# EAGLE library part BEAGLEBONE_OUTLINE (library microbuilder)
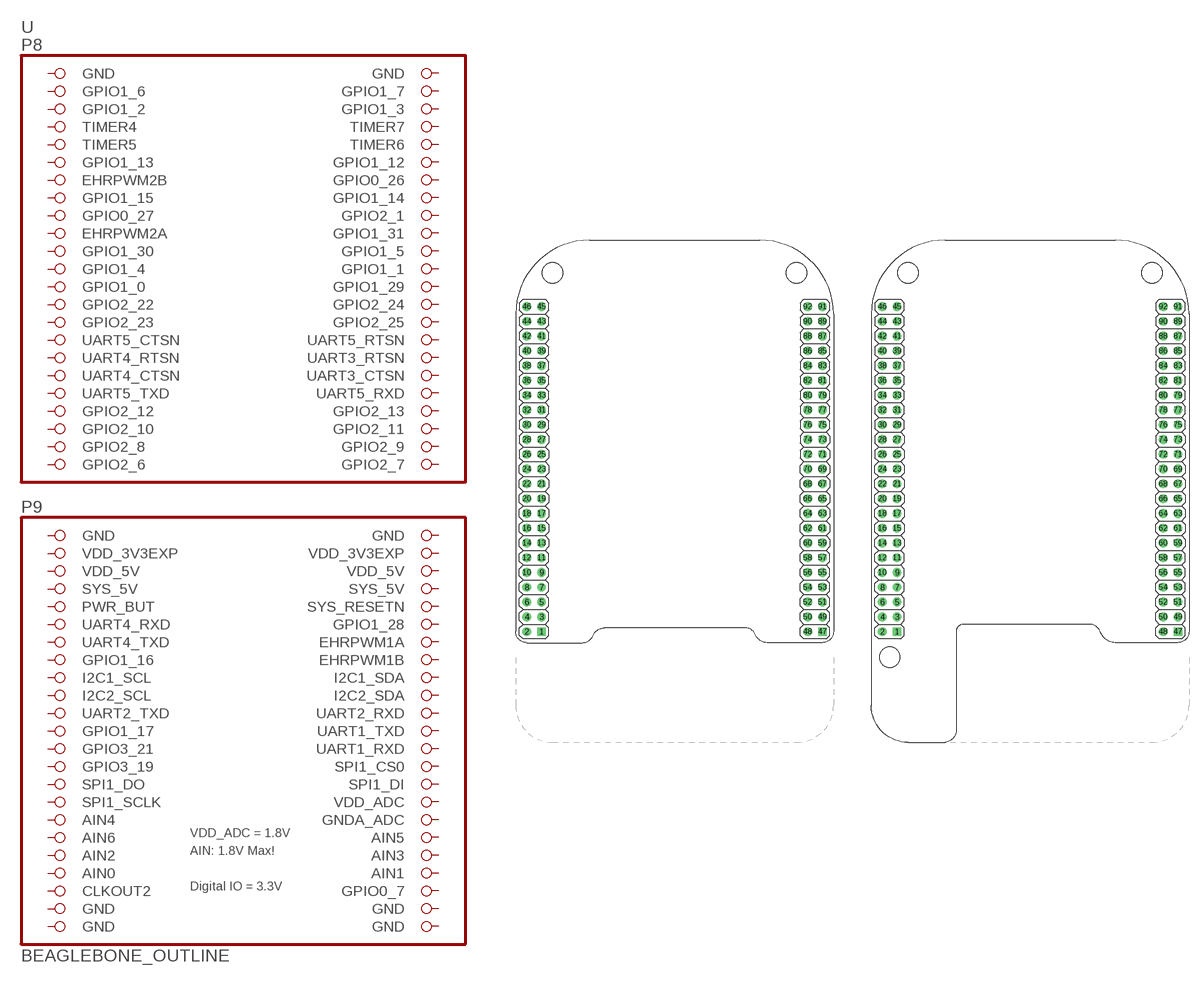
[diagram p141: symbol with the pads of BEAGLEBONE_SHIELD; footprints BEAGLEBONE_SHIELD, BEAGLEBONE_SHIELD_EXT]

Designator prefix -

## BEAGLEBONE_OUTLINE  [BEAGLEBONE_SHIELD]
1  GND  pwr
2  GND  pwr
3  GPIO1_6
4  GPIO1_7
5  GPIO1_2
6  GPIO1_3
7  TIMER4
8  TIMER7
9  TIMER5
10  TIMER6
11  GPIO1_13
12  GPIO1_12
13  EHRPWM2B
14  GPIO0_26
15  GPIO1_15
16  GPIO1_14
17  GPIO0_27
18  GPIO2_1
19  EHRPWM2A
20  GPIO1_31
21  GPIO1_30
22  GPIO1_5
23  GPIO1_4
24  GPIO1_1
25  GPIO1_0
26  GPIO1_29
27  GPIO2_22
28  GPIO2_24
29  GPIO2_23
30  GPIO2_25
31  UART5_CTSN
32  UART5_RTSN
33  UART4_RTSN
34  UART3_RTSN
35  UART4_CTSN
36  UART3_CTSN
37  UART5_TXD  out
38  UART5_RXD  in
39  GPIO2_12
40  GPIO2_13
41  GPIO2_10
42  GPIO2_11
43  GPIO2_8
44  GPIO2_9
45  GPIO2_6
46  GPIO2_7
47  GND  pwr
48  GND  pwr
49  VDD_3V3EXP  pwr
50  VDD_3V3EXP  pwr
51  VDD_5V  pwr
52  VDD_5V  pwr
53  SYS_5V  pwr
54  SYS_5V  pwr
55  PWR_BUT
56  SYS_RESETN  in
57  UART4_RXD  in
58  GPIO1_28
59  UART4_TXD  out
60  EHRPWM1A
61  GPIO1_16
62  EHRPWM1B
63  I2C1_SCL
64  I2C1_SDA
65  I2C2_SCL
66  I2C2_SDA
67  UART2_TXD  out
68  UART2_RXD  in
69  GPIO1_17
70  UART1_TXD  out
71  GPIO3_21
72  UART1_RXD  in
73  GPIO3_19
74  SPI1_CS0
75  SPI1_DO
76  SPI1_DI
77  SPI1_SCLK
78  VDD_ADC  pwr
79  AIN4  in
80  GNDA_ADC  pwr
81  AIN6  in
82  AIN5  in
83  AIN2  in
84  AIN3  in
85  AIN0  in
86  AIN1  in
87  CLKOUT2  out
88  GPIO0_7
89  GND  pwr
90  GND  pwr
91  GND  pwr
92  GND  pwr

## BEAGLEBONE_OUTLINEEXT  [BEAGLEBONE_SHIELD_EXT]
Pads as for BEAGLEBONE_SHIELD

## Footprint BEAGLEBONE_SHIELD (pad centres in mm)
drill 1 square: 1 4.445,19.05; 47 52.705,19.05
drill 1: 2 1.905,19.05; 3 4.445,21.59; 4 1.905,21.59; 5 4.445,24.13; 6 1.905,24.13; 7 4.445,26.67; 8 1.905,26.67; 9 4.445,29.21; 10 1.905,29.21; 11 4.445,31.75; 12 1.905,31.75; 13 4.445,34.29; 14 1.905,34.29; 15 4.445,36.83; 16 1.905,36.83; 17 4.445,39.37; 18 1.905,39.37; 19 4.445,41.91; 20 1.905,41.91; 21 4.445,44.45; 22 1.905,44.45; 23 4.445,46.99; 24 1.905,46.99; 25 4.445,49.53; 26 1.905,49.53; 27 4.445,52.07; 28 1.905,52.07; 29 4.445,54.61; 30 1.905,54.61; 31 4.445,57.15; 32 1.905,57.15; 33 4.445,59.69; 34 1.905,59.69; 35 4.445,62.23; 36 1.905,62.23; 37 4.445,64.77; 38 1.905,64.77; 39 4.445,67.31; 40 1.905,67.31; 41 4.445,69.85; 42 1.905,69.85; 43 4.445,72.39; 44 1.905,72.39; 45 4.445,74.93; 46 1.905,74.93; 48 50.165,19.05; 49 52.705,21.59; 50 50.165,21.59; 51 52.705,24.13; 52 50.165,24.13; 53 52.705,26.67; 54 50.165,26.67; 55 52.705,29.21; 56 50.165,29.21; 57 52.705,31.75; 58 50.165,31.75; 59 52.705,34.29; 60 50.165,34.29; 61 52.705,36.83; 62 50.165,36.83; 63 52.705,39.37; 64 50.165,39.37; 65 52.705,41.91; 66 50.165,41.91; 67 52.705,44.45; 68 50.165,44.45; 69 52.705,46.99; 70 50.165,46.99; 71 52.705,49.53; 72 50.165,49.53; 73 52.705,52.07; 74 50.165,52.07; 75 52.705,54.61; 76 50.165,54.61; 77 52.705,57.15; 78 50.165,57.15; 79 52.705,59.69; 80 50.165,59.69; 81 52.705,62.23; 82 50.165,62.23; 83 52.705,64.77; 84 50.165,64.77; 85 52.705,67.31; 86 50.165,67.31; 87 52.705,69.85; 88 50.165,69.85; 89 52.705,72.39; 90 50.165,72.39; 91 52.705,74.93; 92 50.165,74.93
hole 3.5 at 6.35,80.71
hole 3.5 at 48.26,80.71

## Footprint BEAGLEBONE_SHIELD_EXT (pad centres in mm)
drill 1 square: 1 4.445,19.05; 47 52.705,19.05
drill 1: 2 1.905,19.05; 3 4.445,21.59; 4 1.905,21.59; 5 4.445,24.13; 6 1.905,24.13; 7 4.445,26.67; 8 1.905,26.67; 9 4.445,29.21; 10 1.905,29.21; 11 4.445,31.75; 12 1.905,31.75; 13 4.445,34.29; 14 1.905,34.29; 15 4.445,36.83; 16 1.905,36.83; 17 4.445,39.37; 18 1.905,39.37; 19 4.445,41.91; 20 1.905,41.91; 21 4.445,44.45; 22 1.905,44.45; 23 4.445,46.99; 24 1.905,46.99; 25 4.445,49.53; 26 1.905,49.53; 27 4.445,52.07; 28 1.905,52.07; 29 4.445,54.61; 30 1.905,54.61; 31 4.445,57.15; 32 1.905,57.15; 33 4.445,59.69; 34 1.905,59.69; 35 4.445,62.23; 36 1.905,62.23; 37 4.445,64.77; 38 1.905,64.77; 39 4.445,67.31; 40 1.905,67.31; 41 4.445,69.85; 42 1.905,69.85; 43 4.445,72.39; 44 1.905,72.39; 45 4.445,74.93; 46 1.905,74.93; 48 50.165,19.05; 49 52.705,21.59; 50 50.165,21.59; 51 52.705,24.13; 52 50.165,24.13; 53 52.705,26.67; 54 50.165,26.67; 55 52.705,29.21; 56 50.165,29.21; 57 52.705,31.75; 58 50.165,31.75; 59 52.705,34.29; 60 50.165,34.29; 61 52.705,36.83; 62 50.165,36.83; 63 52.705,39.37; 64 50.165,39.37; 65 52.705,41.91; 66 50.165,41.91; 67 52.705,44.45; 68 50.165,44.45; 69 52.705,46.99; 70 50.165,46.99; 71 52.705,49.53; 72 50.165,49.53; 73 52.705,52.07; 74 50.165,52.07; 75 52.705,54.61; 76 50.165,54.61; 77 52.705,57.15; 78 50.165,57.15; 79 52.705,59.69; 80 50.165,59.69; 81 52.705,62.23; 82 50.165,62.23; 83 52.705,64.77; 84 50.165,64.77; 85 52.705,67.31; 86 50.165,67.31; 87 52.705,69.85; 88 50.165,69.85; 89 52.705,72.39; 90 50.165,72.39; 91 52.705,74.93; 92 50.165,74.93
hole 3.5 at 6.35,80.71
hole 3.5 at 48.26,80.71
hole 3.5 at 3.175,14.67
